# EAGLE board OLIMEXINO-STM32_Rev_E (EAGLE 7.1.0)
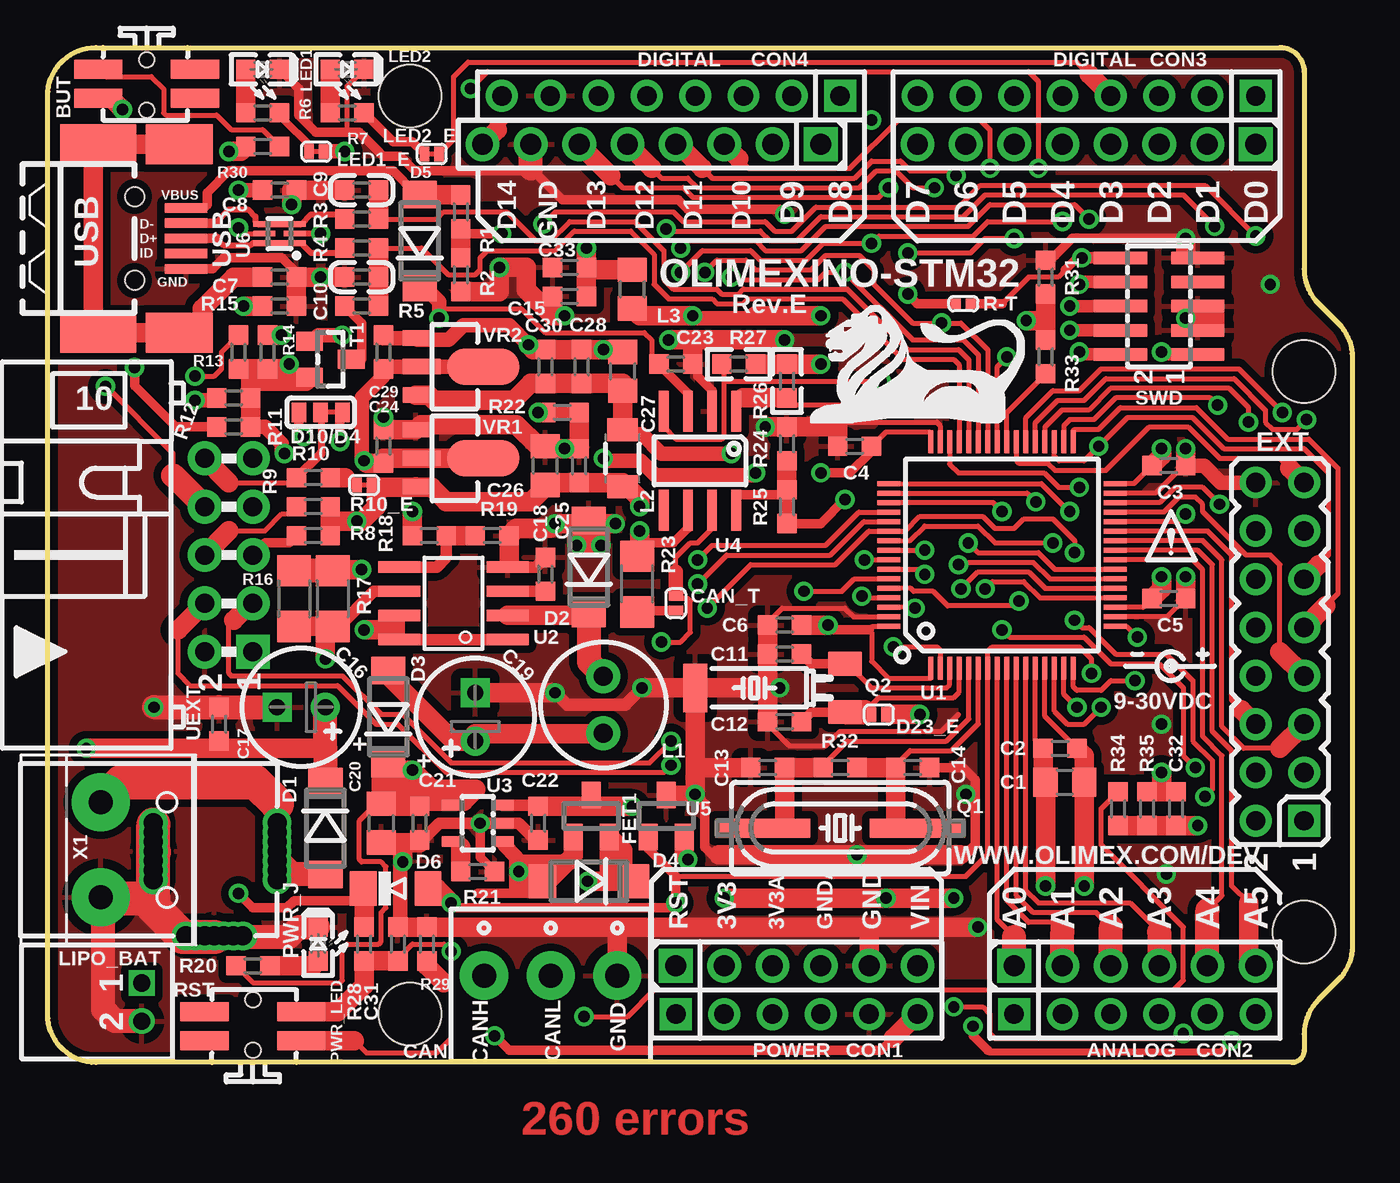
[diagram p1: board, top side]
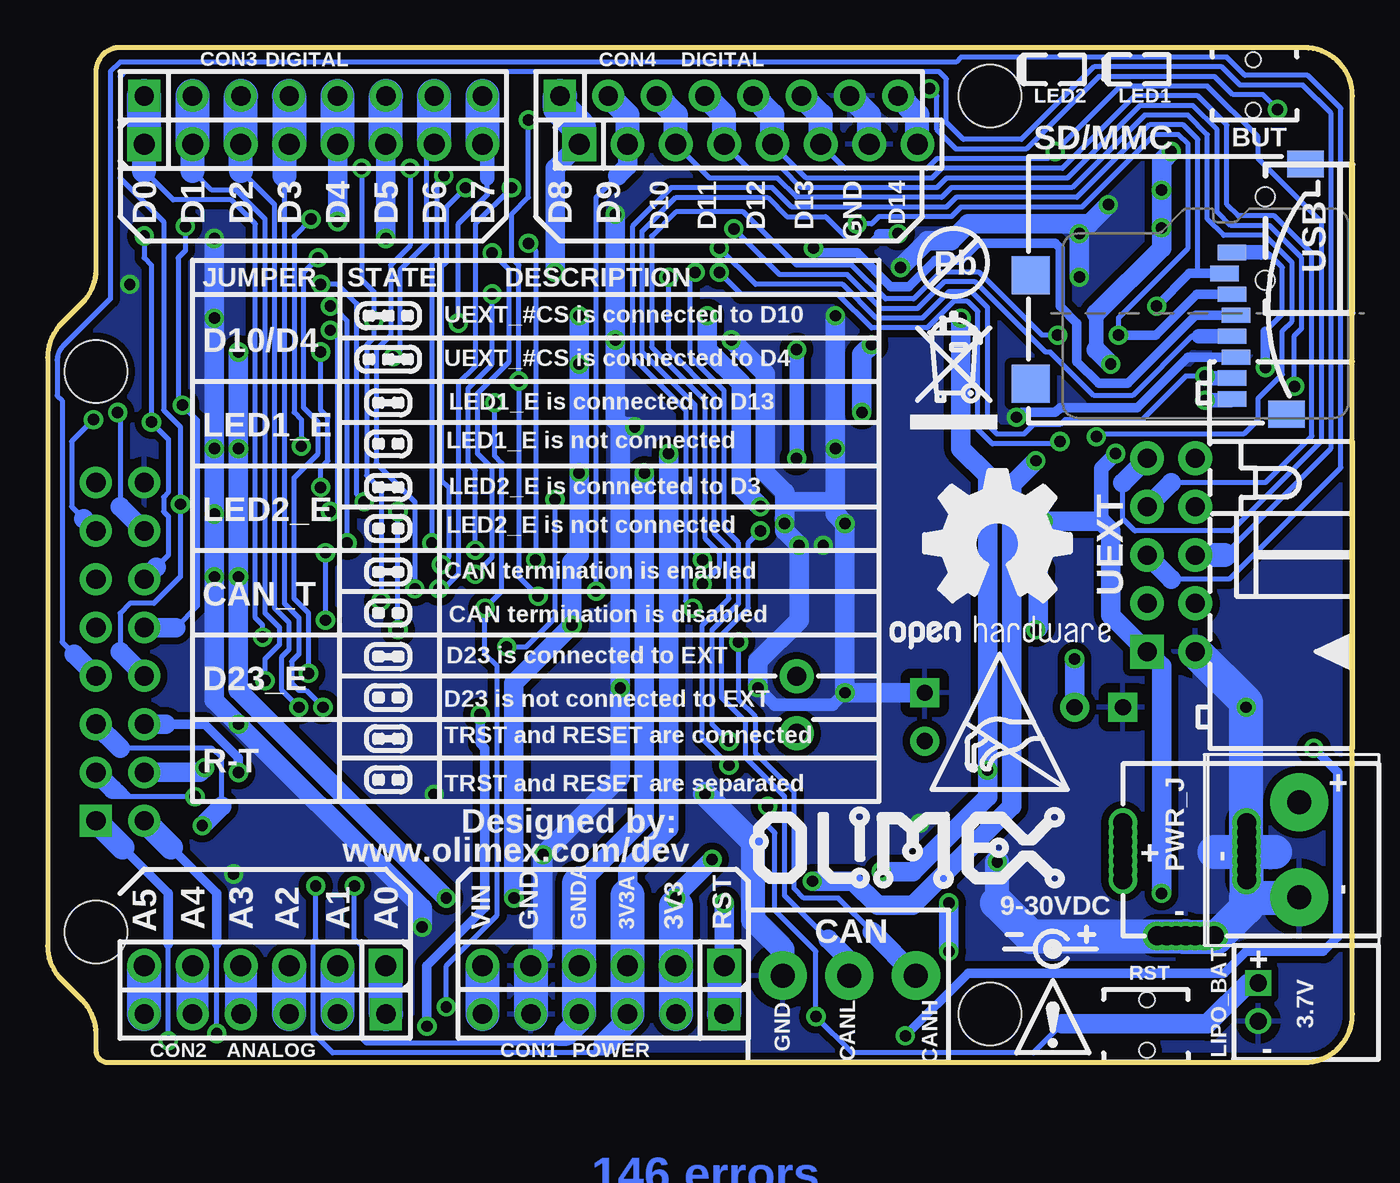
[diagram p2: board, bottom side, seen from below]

Size 68.58 x 53.34 mm. Coordinates in mm from the lower left corner, seen from the top.
Copper layers (1+16): Top 0.035mm / dielectric 1.5mm / Bottom 0.035mm
Design rules "default": minimum track width 10mil, minimum drill 0.6mm, track to track 9.5mil, track to pad 9.5mil, pad to pad 9.5mil, via to via 9.5mil, smd to smd 1mil, copper to edge 10mil, drill to drill 8mil, minimum pad ring 8mil, minimum via ring 8mil, stop-mask expansion 4mil, vias tented up to drill 25mil, thermal gap 20mil
Net classes: 0 default: width 0.241 mm, drill 0.584 mm, clearance 0.241 mm; 1 pwr: width 0.25 mm

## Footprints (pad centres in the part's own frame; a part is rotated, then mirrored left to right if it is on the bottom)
SW_TAKT3X4 = smd 2.54 x 1.016: 1_1 -2.54,0.762; 1_2 2.54,0.762; 2_1 -2.54,-0.762; 2_2 2.54,-0.762 | hole 0.8: 0,-1.397; 0,1.27
C0805_5MIL_DWS = smd 1.27 x 1.524: 1 -1.016,0; 2 1.016,0
C0603_DWS = smd 1.016 x 1.016: 1 -0.889,0; 2 0.889,0
C0603_DWS_NA = smd 1.016 x 1.016: 1 -0.889,0; 2 0.889,0
E2,5-6,3 = drill 0.864 pad 1.524: + -1.27,0 | drill 0.864 pad 1.524 square: - 1.27,0
CON3/3.5MM = drill 1.27 pad 2.54: 1 -1.75,-0.5; 2 1.75,-0.5; 3 5.25,-0.5
SJ_1_SMALLER = smd 0.508 x 0.762: 1 -0.381,0; 2 0.381,0
PN1X6 = drill 1.1 pad 1.778 square: 1 -6.35,0 | drill 1.1 pad 1.778: 2 -3.81,0; 3 -1.27,0; 4 1.27,0; 5 3.81,0; 6 6.35,0
PN1X8 = drill 1.1 pad 1.778 square: 1 -8.89,0 | drill 1.1 pad 1.778: 2 -6.35,0; 3 -3.81,0; 4 -1.27,0; 5 1.27,0; 6 3.81,0; 7 6.35,0; 8 8.89,0
MLL-41 = smd 1.45 x 1.8: A 2.445,0; K -2.445,0
MINI-MELF = smd 1.4 x 1.8: A 1.7,0; C -1.7,0
SJ_2_SMALL = smd 0.762 x 1.016: 1 -1.143,0; 2 0,0; 3 1.143,0
HN2X8-MALE = drill 1.016 pad 1.676 square: 1 -8.89,-1.27 | drill 1.016 pad 1.676: 2 -8.89,1.27; 3 -6.35,-1.27; 4 -6.35,1.27; 5 -3.81,-1.27; 6 -3.81,1.27; 7 -1.27,-1.27; 8 -1.27,1.27; 9 1.27,-1.27; 10 1.27,1.27; 11 3.81,-1.27; 12 3.81,1.27; 13 6.35,-1.27; 14 6.35,1.27; 15 8.89,-1.27; 16 8.89,1.27
SOT23 = smd 1 x 1.4: 1 -0.95,-1.1; 2 0.95,-1.1; 3 0,1.1
SW68 = drill 1 pad 1.778: 1 -1.5,0; 2 1.5,0
L3216C = smd 1.2 x 1.6: 1 -1.5,0; 2 1.5,0
L0805_5MIL_DWS = smd 1.27 x 1.524: 1 -1.016,0; 2 1.016,0
LED-0603 = smd 1.016 x 1.016: A 0.889,0; C -0.889,0
SJ_1_SMALLER_CLOSE = smd 0.508 x 0.762: 1 -0.381,0; 2 0.381,0
DW02R = drill 0.9 square: 1 -1,0 | drill 0.9: 2 1,0
STM32-MAPLE_PATFORM = drill 1.016 pad 1.676: 3V3 35.56,2.54; 3V3A 38.1,2.54; A1 53.34,2.54; A2 55.88,2.54; A3 58.42,2.54; A4 60.96,2.54; A5 63.5,2.54; D1 60.96,50.8; D2 58.42,50.8; D3 55.88,50.8; D4 53.34,50.8; D5 50.8,50.8; D6 48.26,50.8; D7 45.72,50.8; D9 39.116,50.8; D10 36.576,50.8; D11 34.036,50.8; D12 31.496,50.8; D13 28.956,50.8; D14 23.876,50.8; GND 43.18,2.54; GND@1 26.416,50.8; GNDA 40.64,2.54; VIN 45.72,2.54 | drill 1.016 pad 1.676 square: A0 50.8,2.54; D0 63.5,50.8; D8 41.656,50.8; RST 33.02,2.54 | hole 3.3: 66.04,36.322; 66.04,6.858; 19.05,50.8; 19.05,2.54
PWR_JACK_UNI_MILLING = drill 1: + 0,4.75; +1 0,5.25; +2 0,5.75; +3 0,6.25; +4 0,4.25; +5 0,3.75; +6 0,3.25; - -6.5,4.75; -1 -6.5,5.25; -2 -6.5,5.75; -3 -6.5,4.25; -4 -6.5,3.75; -5 -6.5,6.25; -6 -6.5,3.25; -- -3.3,0.3; --1 -3.8,0.3; --2 -4.3,0.3; --3 -4.8,0.3; --4 -2.8,0.3; --5 -2.3,0.3; --6 -1.8,0.3
HC49/SMD2_THIN = smd 5 x 1: 1 -4.064,0; 2 4.064,0
TC26H_3_REPAIR_SMD = smd 1.27 x 1.778: 1 -1.27,0; 2 1.27,0 | smd 2.54 x 1.27: GND 0,7.874
R0603_5MIL_DWS = smd 1.016 x 1.016: 1 -0.889,0; 2 0.889,0
R1206_5MIL_WS = smd 1.651 x 1.778: 1 -1.46,0; 2 1.46,0
0603_0R = smd 1.016 x 1.016: 1 -0.889,0; 2 0.889,0
R0603_5MIL_DWS_NA = smd 1.016 x 1.016: 1 -0.889,0; 2 0.889,0
SJ_1_THE_SMALLEST = smd 0.508 x 0.508: 1 -0.381,0; 2 0.381,0
TFR-MEM-CON = smd 0.8 x 1.5: 1 -3.2,10.7; 2 -2.1,10.3; 3 -1,10.7; 4 0.1,10.9; 5 1.2,10.7; 6 2.3,10.9; 7 3.4,10.7; 8 4.5,10.7 | smd 2 x 2: 9 3.7,0.1; 10 -2,0.1 | smd 1.4 x 1.9: 11 5.3,13.55; 12 -7.85,14.55
ML10_50MILS_M = smd 0.66 x 2.794: 1 -2.54,-2.032; 2 -2.54,2.032; 3 -1.27,-2.032; 4 -1.27,2.032; 5 0,-2.032; 6 0,2.032; 7 1.27,-2.032; 8 1.27,2.032; 9 2.54,-2.032; 10 2.54,2.032
SOT-23 = smd 1 x 1.4: 1 -0.95,-1.1; 2 0.95,-1.1; 3 0,1.1
LPTQFP64 = smd 1.2 x 0.254: 1 -5.95,3.75; 2 -5.95,3.25; 3 -5.95,2.75; 4 -5.95,2.25; 5 -5.95,1.75; 6 -5.95,1.25; 7 -5.95,0.75; 8 -5.95,0.25; 9 -5.95,-0.25; 10 -5.95,-0.75; 11 -5.95,-1.25; 12 -5.95,-1.75; 13 -5.95,-2.25; 14 -5.95,-2.75; 15 -5.95,-3.25; 16 -5.95,-3.75; 33 5.95,-3.75; 34 5.95,-3.25; 35 5.95,-2.75; 36 5.95,-2.25; 37 5.95,-1.75; 38 5.95,-1.25; 39 5.95,-0.75; 40 5.95,-0.25; 41 5.95,0.25; 42 5.95,0.75; 43 5.95,1.25; 44 5.95,1.75; 45 5.95,2.25; 46 5.95,2.75; 47 5.95,3.25; 48 5.95,3.75 | smd 0.254 x 1.2: 17 -3.75,-5.95; 18 -3.25,-5.95; 19 -2.75,-5.95; 20 -2.25,-5.95; 21 -1.75,-5.95; 22 -1.25,-5.95; 23 -0.75,-5.95; 24 -0.25,-5.95; 25 0.25,-5.95; 26 0.75,-5.95; 27 1.25,-5.95; 28 1.75,-5.95; 29 2.25,-5.95; 30 2.75,-5.95; 31 3.25,-5.95; 32 3.75,-5.95; 49 3.75,5.95; 50 3.25,5.95; 51 2.75,5.95; 52 2.25,5.95; 53 1.75,5.95; 54 1.25,5.95; 55 0.75,5.95; 56 0.25,5.95; 57 -0.25,5.95; 58 -0.75,5.95; 59 -1.25,5.95; 60 -1.75,5.95; 61 -2.25,5.95; 62 -2.75,5.95; 63 -3.25,5.95; 64 -3.75,5.95
SO-8 = smd 0.6 x 2.2: 1 -1.905,-2.854; 2 -0.635,-2.854; 3 0.635,-2.854; 4 1.905,-2.854; 5 1.905,2.854; 6 0.635,2.854; 7 -0.635,2.854; 8 -1.905,2.854
SOT-23-5 = smd 0.55 x 1.2: 1 -0.95,-1.3; 2 0,-1.3; 3 0.95,-1.3; 4 0.95,1.3; 5 -0.95,1.3
SO-08_THIN = smd 0.508 x 2.159: 1 -1.905,-2.603; 2 -0.635,-2.603; 3 0.635,-2.603; 4 1.905,-2.603; 5 1.905,2.603; 6 0.635,2.603; 7 -0.635,2.603; 8 -1.905,2.603
USBLC6-2P6 = smd 0.3 x 1.46: 1 -0.5,-0.65; 3 0.5,-0.65; 4 0.5,0.65; 6 -0.5,0.65 | smd 0.3 x 1.16: 2 0,-0.8; 5 0,0.8
BH10R = drill 1 pad 1.778 square: 1 -5.08,-1.27 | drill 1 pad 1.778: 2 -5.08,1.27; 3 -2.54,-1.27; 4 -2.54,1.27; 5 0,-1.27; 6 0,1.27; 7 2.54,-1.27; 8 2.54,1.27; 9 5.08,-1.27; 10 5.08,1.27
USB_MINI_9PIN = smd 2.25 x 0.5: D+ 2.706,0; D- 2.706,0.8; GND 2.706,-1.6; ID 2.706,-0.8; VBUS 2.706,1.6 | smd 4 x 2.1: GND1 -1.9,4.95; GND3 -1.9,-4.95 | smd 3.5 x 2.1: GND2 2.35,4.95; GND4 2.35,-4.95 | hole 1: 0,2.2; 0,-2.2
SOT89_REP_THERMALOFF = smd 0.8 x 1.4: 1 -1.499,-1.981; 3 1.499,-1.981 | smd 0.8 x 2: 2 0,-1.681 | smd 1.93 x 3.81: P$2 0,1.57
W237-102 = drill 1.27 pad 3.048: 1 -2.5,-1.27; 2 2.5,-1.27

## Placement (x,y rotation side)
BUT  SW-SIDE_WTCM-TR(3X4)  [SW_TAKT3X4]  5.21,51.44 0 top
C1  10uF/6.3V  [C0805_5MIL_DWS]  53.47,14.73 0 top
C2  100nF  [C0603_DWS]  53.21,16.51 0 top
C3  100nF  [C0603_DWS]  58.93,31.37 180 top
C4  100nF  [C0603_DWS]  42.42,32.38 0 top
C5  100nF  [C0603_DWS]  58.93,24.38 180 top
C6  4.7uF/6.3V  [C0603_DWS]  38.73,22.99 0 top
C7  10nF  [C0603_DWS]  12.19,41.27 0 top
C8  100nF  [C0603_DWS]  12.19,45.85 180 top
C9  NA(47pF)  [C0603_DWS_NA]  16.51,45.85 180 top
C10  NA(47pF)  [C0603_DWS_NA]  16.51,41.27 180 top
C11  10pF  [C0603_DWS]  38.73,21.46 180 top
C12  10pF  [C0603_DWS]  38.73,17.91 180 top
C13  27pF  [C0603_DWS]  37.85,15.49 180 top
C14  27pF  [C0603_DWS]  45.47,15.49 0 top
C15  22uF/6.3V  [C0603_DWS]  27.43,40.26 180 top
C16  CE 100uF/35V/6.3x11mm/RM2.5  [E2,5-6,3]  13.34,18.67 180 top
C17  100nF  [C0603_DWS]  9.02,17.78 90 top
C18  820pF  [C0603_DWS]  26.16,25.65 90 top
C19  CE 470uF/10V/6.3x11mm/RM2.5  [E2,5-6,3]  22.48,18.16 90 top
C20  10uF/6.3V  [C0805_5MIL_DWS]  17.53,12.57 270 top
C21  2.2uF  [C0603_DWS]  19.56,12.57 270 top
C22  2.2uF  [C0603_DWS]  25.78,12.57 270 top
C23  100nF  [C0603_DWS]  33.02,36.7 0 top
C24  2.2uF  [C0603_DWS]  17.65,32.38 90 top
C25  100nF  [C0603_DWS]  27.94,31.37 90 top
C26  10uF/6.3V  [C0805_5MIL_DWS]  26.16,31.37 90 top
C27  10uF/6.3V  [C0805_5MIL_DWS]  30.23,36.32 90 top
C28  10nF  [C0603_DWS]  28.07,36.58 90 top
C29  2.2uF  [C0603_DWS]  17.65,37.34 90 top
C30  2.2uF  [C0603_DWS]  26.16,36.58 90 top
C31  100nF  [C0603_DWS]  18.41,6.22 90 top
C32  10nF  [C0603_DWS]  59.31,13.34 270 top
C33  22uF/6.3V  [C0603_DWS]  27.43,41.78 180 top
CAN  TB3-3.5MM  [CON3/3.5MM]  28.19,4.06 180 top
CAN_T  Open  [SJ_1_SMALLER]  33.02,24.13 90 top
CON1  NA  [PN1X6]  39.37,5.08 0 top
CON2  NA  [PN1X6]  57.15,5.08 0 top
CON3  NA  [PN1X8]  54.61,48.26 180 top
CON4  NA  [PN1X8]  31.75,48.26 180 top
D1  1N5819S/SS14  [MLL-41]  14.61,12.32 270 top
D2  1N5819S/SS14  [MLL-41]  28.45,26.04 90 top
D3  1N5819S/SS14  [MLL-41]  17.91,18.16 90 top
D4  1N5819S/SS14  [MLL-41]  28.45,9.53 180 top
D5  1N5819S/SS14  [MLL-41]  19.56,43.18 90 top
D6  1N4148/mini-melf  [MINI-MELF]  18.29,9.14 0 top
D10/D4  D10:Open/D4:Close  [SJ_2_SMALL]  14.35,34.16 180 top
D23_E  Open  [SJ_1_SMALLER]  43.69,18.29 0 top
EXT  PN2x8  [HN2X8-MALE]  64.77,21.59 90 top
FET1  IRLML6402  [SOT23]  28.57,12.95 0 top
L1  CL10uH SW68  [SW68]  29.21,18.8 270 top
L2  NA  [L3216C]  30.23,31.75 90 top
L3  CL470nH/0805/1.76R/250mA  [L0805_5MIL_DWS]  30.73,40.64 90 top
LED1  GREEN(0603)  [LED-0603]  11.3,52.2 180 top
LED1_E  Close  [SJ_1_SMALLER_CLOSE]  14.12,47.88 0 top
LED2  YELLOW(0603)  [LED-0603]  15.75,52.2 180 top
LED2_E  Close  [SJ_1_SMALLER_CLOSE]  20.19,47.75 0 top
LIPO_BAT  DW02R  [DW02R]  4.95,3.17 270 top
PLATFORM1  STM32-MAPLE_PLATFORM  [STM32-MAPLE_PATFORM]  0,0 0 top
PWR_J  YDJ-1136  [PWR_JACK_UNI_MILLING]  12.06,6.35 0 top
PWR_LED  RED(0603)  [LED-0603]  14.22,6.22 270 top
Q1  Q8.000MHz/20pF/HC-49SM(SMD)  [HC49/SMD2_THIN]  41.66,12.32 180 top
Q2  32768Hz/6pF  [TC26H_3_REPAIR_SMD]  41.91,19.68 90 top
R1  15k  [R0603_5MIL_DWS]  21.72,44.7 270 top
R2  22k  [R0603_5MIL_DWS]  21.72,41.4 270 top
R3  22R  [R0603_5MIL_DWS]  16.51,44.32 180 top
R4  22R  [R0603_5MIL_DWS]  16.51,42.8 180 top
R5  1.5k  [R0603_5MIL_DWS]  16.51,39.75 180 top
R6  2k  [R0603_5MIL_DWS]  11.3,49.91 0 top
R7  2k  [R0603_5MIL_DWS]  15.75,49.91 0 top
R8  4.7k  [R0603_5MIL_DWS]  13.97,27.69 0 top
R9  4.7k  [R0603_5MIL_DWS]  13.97,29.21 0 top
R10  10k  [R0603_5MIL_DWS]  13.97,30.73 0 top
R10_E  Close  [SJ_1_SMALLER_CLOSE]  16.64,30.35 0 top
R11  100k  [R0603_5MIL_DWS]  9.78,33.4 180 top
R12  100k  [R0603_5MIL_DWS]  9.78,34.92 180 top
R13  100k  [R0603_5MIL_DWS]  10.03,37.34 90 top
R14  10k  [R0603_5MIL_DWS]  11.56,37.34 90 top
R15  1M  [R0603_5MIL_DWS]  12.19,39.75 180 top
R16  0.47R  [R1206_5MIL_WS]  12.95,24.38 90 top
R17  0.47R  [R1206_5MIL_WS]  14.99,24.38 90 top
R18  3.01k/1%  [R0603_5MIL_DWS]  20.07,27.69 0 top
R19  1k/1%  [R0603_5MIL_DWS]  23.37,27.69 0 top
R20  2k  [R0603_5MIL_DWS]  10.79,5.08 0 top
R21  15k  [R0603_5MIL_DWS]  22.61,10.03 180 top
R22  0R(boad mounted)  [0603_0R]  27.05,34.16 180 top
R23  120R  [R1206_5MIL_WS]  30.99,25.15 270 top
R24  10k  [R0603_5MIL_DWS]  38.86,32.51 270 top
R25  0R(boad mounted)  [0603_0R]  38.86,29.21 90 top
R26  NA(4.7k)  [R0603_5MIL_DWS_NA]  38.86,35.81 270 top
R27  NA(4.7k)  [R0603_5MIL_DWS_NA]  36.32,36.7 180 top
R28  10k  [R0603_5MIL_DWS]  16.64,6.22 270 top
R29  330R  [R0603_5MIL_DWS]  19.94,6.22 270 top
R30  1k  [R0603_5MIL_DWS]  11.3,48.13 0 top
R31  10k  [R0603_5MIL_DWS]  52.45,41.27 90 top
R32  1M  [R0603_5MIL_DWS]  41.66,15.49 180 top
R33  1k  [R0603_5MIL_DWS]  52.45,37.08 270 top
R34  3M  [R0603_5MIL_DWS]  56.26,13.34 90 top
R35  1M  [R0603_5MIL_DWS]  57.78,13.34 90 top
R-T  Open  [SJ_1_THE_SMALLEST]  48.13,39.88 0 top
RST  SW-SIDE_WTCM-TR(3X4)  [SW_TAKT3X4]  10.79,1.91 180 top
SD/MMC  MICRO  [TFR-MEM-CON]  17.02,39.37 270 bottom
SWD  GPH127SMT-02x05(PIN7-CUT)  [ML10_50MILS_M]  58.42,39.75 90 top
T1  DTA114YKA  [SOT-23]  14.86,36.96 270 top
U1  STM32F103RBT6(LQFP64)  [LPTQFP64]  50.16,26.67 90 top
U2  MC33063ADR(SO8)  [SO-8]  21.34,24.13 90 top
U3  MCP73812T-420I/OT  [SOT-23-5]  22.61,12.57 90 top
U4  MCP2551-I/SN  [SO-08_THIN]  34.29,31.62 180 top
U5  NA  [SOT23]  32.51,12.95 0 top
U6  NA  [USBLC6-2P6]  12.19,43.56 90 top
U$1  [LION_12X7MM]  45.34,35.18 0 top
U$5  [PB_SMALL]  20.95,42.04 0 bottom
U$6  [RECYCLE_BIN1/8]  23.24,33.27 0 bottom
U$7  [ESD_SYMBOL]  22.1,14.35 0 bottom
U$8  [ATTENTION_SMALL]  57.78,26.4 0 top
U$9  [OLIMEX1_V]  13.97,9.02 0 bottom
U$10  [ROHS]  not placed on the board
U$11  [LOGO-OPENHARDWARE_8X8]  18.67,27.18 0 bottom
U$12  [ATTENTION]  17.65,0.51 0 bottom
UEXT  BH10R  [BH10R]  9.53,26.67 90 top
USB  USB-MINI  [USB_MINI_9PIN]  4.57,43.31 0 top
VR1  MCP1700T-3302E/MB  [SOT89_REP_THERMALOFF]  21.34,31.75 270 top
VR2  MCP1700T-3302E/MB  [SOT89_REP_THERMALOFF]  21.34,36.58 270 top
X1  NA  [W237-102]  4.06,11.18 270 top

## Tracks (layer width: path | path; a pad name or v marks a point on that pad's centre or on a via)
+5V  (via drill 0.6)
  Top 0.254: R20.1 10.79,4.19 15.37,4.19 15.49,4.32 15.49,5.97 15.75,6.22 17.4,6.22 17.53,6.35 17.53,7.87 17.78,8.13 17.78,10.29 17.53,10.54 16.51,10.54 16.38,10.67 16.38,12.7 17.27,13.59 C20.1 | C23.1 31.75,37.08 31.75,37.97 31.37,38.35 26.16,38.35 24.89,39.62 20.57,39.62
  Top 0.508: U4.3 33.66,35.18 C23.1 | 22.61,8.89 24.86,8.89 24.86,9.14
  Top 0.559: U3.1 23.91,11.53 24,11.43
  Top 0.61: U3.4 19.56,13.52 C21.1
  Top 0.762: v24.77,10.03 24.64,10.03 24.64,10.54 | 24,11.43 24.64,10.79 24.64,10.54 | v20.57,39.12 20.57,39.62 20.57,39.97 19.81,40.73 D5.K | 24.64,10.54 27.3,10.54
  Top 1.016: v19.18,28.96 R18.1 | 17.91,15.37 D3.K 17.91,15.49 | 17.91,15.37 v19.18,15.37 20.32,14.22 | 17.53,13.72 C20.1 17.53,13.46 C21.1 19.56,13.72 17.53,13.72 | FET1.1 27.62,10.86 27.3,10.54 26.29,9.53 D4.A 26,10.03 v24.77,10.03 24.77,9.14 24.86,9.14 26,9.14 | 17.53,13.72 21.87,13.72 22.5,14.35 17.91,14.35 17.91,15.37 | 17.53,13.72 17.53,15.49 17.91,15.49 | 17.91,15.49 17.91,15.37
  Bottom 1.016: v24.77,10.03 23.11,10.03 19.18,13.97 v19.18,15.37 v19.18,28.96 19.18,30.86 20.57,32.26 v20.57,39.12
+5V_USB
  Top 0.508: USB.VBUS 8.2,44.91 8.38,45.09 8.38,45.72 9.53,46.86 18.16,46.86 19.3,45.72 19.56,45.72
  Top 0.762: 19.56,45.72 19.56,45.59
  Top 1.016: D5.A 19.56,45.59 R1.1
+24V  (via drill 0.6)
  Top 0.508: v23.5,1.4 24.26,0.64 43.81,0.64 44.45,1.27
  Top 0.61: U2.6 17.14,24.77 15.24,22.86 15.24,22.73
  Top 1.016: R17.1 14.99,22.73 | v14.61,21.21 14.61,22.73 15.24,22.73 15.24,22.67 R17.1 | R17.1 R16.1 | v2.03,16.51 9.02,16.51 | 9.02,16.51 14.61,16.51 | 44.45,1.27 PLATFORM1.VIN | 9.02,16.51 C17.1
  Top 1.27: D1.K 14.61,16.51 C16.+
  Bottom 0.508: v2.03,16.51 0.76,15.24 0.76,6.6 1.52,5.84 5.59,5.84 6.73,4.7 20.19,4.7 v23.5,1.4
  Bottom 1.016: C16.+ v14.61,21.21
  Bottom 1.778: PLATFORM1.VIN CON1.6
AGND  (via drill 0.6)
  Top 0.254: U1.12 51.91,16.92 C2.1
  Top 0.762: v37.21,30.99 37.21,30.86 31.93,30.86 31.17,31.62 29.21,31.62 v29.21,31.75 | C29.2 17.65,38.08 VR2.1 19.46,37.97 21.08,37.97 21.84,38.73 24.26,38.73 v25.27,37.72 | R22.2 28.07,34.16
  Top 1.016: C2.1 52.32,14.73 C1.1 v52.45,9.27 | C27.2 30.23,37.47 v29.21,37.47 C28.2 C30.2 25.53,37.47 v25.27,37.72 | v25.78,34.16 R22.2
  Bottom 0.254: 41.27,1.52 41.27,1.02 41.78,1.02 | 41.78,1.02 51.82,1.02 52.07,1.27 52.07,6.1 52.45,6.48 v52.45,9.27 | 41.78,1.02 41.78,1.52
  Bottom 0.762: v29.21,31.75 v29.21,37.47
  Bottom 1.016: 40.64,9.4 37.21,12.83 v37.21,30.99 | v25.27,37.72 25.78,37.21 v25.78,34.16
  Bottom 1.27: 41.27,1.52 40.64,2.16 PLATFORM1.GNDA
  Bottom 1.778: PLATFORM1.GNDA CON1.4 40.64,9.4
BOOT0  (via drill 0.6)
  Top 0.254: U1.60 45.37,24.92 45.52,24.77 46.54,24.77 47.3,24 50.8,24 v51.05,24.26 | v52.07,46.99 52.07,51.56 51.56,52.07 23.11,52.07 v22.23,51.18
  Top 1.016: 52.45,38.99 R33.1 | BUT.2_1 3.35,50.67 v3.94,50.09 | v51.44,38.99 52.45,38.99 | 52.45,38.99 R31.1
  Bottom 0.254: v51.05,24.26 51.05,30.1 51.82,30.86 51.82,37.72 51.44,38.1 v51.44,38.99 51.44,40.51 52.07,41.15 v52.07,46.99 | v3.94,50.09 4.71,50.86 6.29,50.86 7.24,51.82 13.34,51.82 17.14,48.01 20.83,48.01 21.84,49.02 21.84,50.8 v22.23,51.18
D0(RXD2)  (via drill 0.6)
  Top 0.254: U1.17 56.71,22.92 v57.28,22.35
  Bottom 0.254: v57.28,22.35 57.28,22.99 57.66,23.37 57.66,44.07 58.93,45.34 61.98,45.34 63.5,46.86
  Bottom 1.27: 63.5,46.86 CON3.1
  Bottom 1.778: CON3.1 PLATFORM1.D0
D1(TXD2)  (via drill 0.6)
  Top 0.254: U1.16 53.91,19.75 54.1,19.56 55.37,19.56 55.88,20.07 v57.15,20.07
  Bottom 0.254: v57.15,20.07 57.15,21.21 56.39,21.97 56.39,22.86 57.15,23.62 57.15,44.32 58.67,45.85 59.94,45.85 60.96,46.86
  Bottom 1.27: 60.96,46.86 CON3.2
  Bottom 1.778: CON3.2 PLATFORM1.D1
D2  (via drill 0.6)
  Top 0.254: U1.14 52.91,18.46 53.59,17.78 54.48,17.78 v55.37,18.67
  Bottom 0.254: v55.37,18.67 56.26,19.56 56.26,21.34 55.88,21.72 55.88,23.11 56.64,23.88 56.64,45.09 58.42,46.86
  Bottom 1.27: 58.42,46.86 CON3.3
  Bottom 1.778: CON3.3 PLATFORM1.D2
D3(LED2)  (via drill 0.6)
  Top 0.254: U1.15 53.41,19.36 v54.1,18.67 | LED2_E.2 21.34,48.51 21.34,51.82 22.1,52.58 54.1,52.58 54.74,51.94
  Top 1.016: 54.74,51.94 PLATFORM1.D3
  Bottom 0.254: v54.1,18.67 54.99,19.56 55.37,19.56 55.75,19.94 55.75,21.08 55.37,21.46 55.37,23.37 56.13,24.13 56.13,46.61
  Bottom 1.27: 56.13,46.61 56.13,48.01 CON3.4
  Bottom 1.778: PLATFORM1.D3 CON3.4
D4  (via drill 0.6)
  Top 0.254: v42.93,26.42 U1.57 | v53.34,44.2 49.4,44.2 48.64,43.43 43.69,43.43 v43.31,43.05 40.77,43.05 39.88,42.16 37.47,42.16 36.96,42.67 34.42,42.67 v33.27,41.53 | 15.37,34.16 14.35,34.16
  Top 0.508: v15.37,32.64 15.37,34.16 D10/D4.1
  Bottom 0.254: v42.93,26.42 42.93,42.67 v43.31,43.05 | v15.37,32.64 15.49,32.51 18.92,32.51 19.68,33.27 19.68,39.47 20.22,40.01 20.95,40.01 22.35,38.61 25.27,38.61 27.05,40.39 32.13,40.39 v33.27,41.53
  Bottom 1.016: v53.34,44.2 CON3.5
  Bottom 1.778: CON3.5 PLATFORM1.D4
D5  (via drill 0.6)
  Top 0.254: U1.58 45.84,25.92 v46.1,25.65 | v45.21,42.55 48.51,42.55 49.28,43.31 v50.8,43.31
  Bottom 0.254: v46.1,25.65 45.21,26.54 45.21,31.24 45.97,32 45.97,35.18 44.32,36.83 44.32,41.66 v45.21,42.55
  Bottom 1.016: v50.8,43.31 CON3.6
  Bottom 1.778: CON3.6 PLATFORM1.D5
D6  (via drill 0.6)
  Top 0.254: U1.41 49.91,36.57 v50.42,37.08
  Bottom 0.254: v50.42,37.08 50.04,37.47 50.04,41.66 48.64,43.05 48.64,47.88 CON3.7
  Bottom 1.778: CON3.7 PLATFORM1.D6
D7(TXD1)  (via drill 0.6)
  Top 0.254: U1.42 49.41,37.45 48.01,38.86 v46.99,38.86 45.47,38.86 43.43,40.89 43.43,41.66 42.67,42.42 40.89,42.42 40.13,41.66 37.21,41.66 36.7,42.16 35.18,42.16 v34.54,41.53 | v32.77,16.89 31.62,15.75 21.21,15.75 18.67,18.29 17.53,18.29 15.49,20.32 9.65,20.32 9.53,20.45 9.53,22.99 9.78,23.24
  Top 1.016: 9.78,23.24 10.67,24.13 UEXT.3
  Bottom 0.254: v46.99,38.86 46.99,44.07 45.47,45.59 45.47,46.48 | v34.54,41.53 34.8,41.27 34.8,37.08 33.02,35.31 33.02,28.07 32.26,27.3 32.26,24.13 33.66,22.73 33.66,17.78 v32.77,16.89
  Bottom 0.508: 45.47,48.01 CON3.8
  Bottom 0.762: 45.47,46.48 45.47,48.01
  Bottom 1.778: CON3.8 PLATFORM1.D7
D8(RXD1)  (via drill 0.6)
  Top 0.254: U1.43 48.91,37.19 48.13,37.97 45.47,37.97 v41.91,41.53 40.89,41.53 40.51,41.15 36.07,41.15 v35.94,41.27 | v32.77,15.62 32.38,15.24 20.95,15.24 18.41,17.78 17.27,17.78 15.24,19.81 7.49,19.81 6.86,20.45 6.86,22.73
  Top 1.016: 6.86,22.73 UEXT.4
  Bottom 0.254: v35.94,41.27 35.94,37.47 33.53,35.05 33.53,27.81 32.77,27.05 32.77,24.38 34.16,22.99 34.16,17.02 v32.77,15.62
  Bottom 1.016: v41.91,41.53 41.91,46.99 CON4.1
  Bottom 1.778: CON4.1 40.64,49.15 41.66,50.16 PLATFORM1.D8
D9  (via drill 0.6)
  Top 0.254: U1.59 42.4,25.42 41.74,24.77 v39.75,24.77
  Bottom 0.254: v39.75,24.77 39.75,45.47 38.61,46.61
  Bottom 1.016: 38.61,46.61 38.1,47.12 CON4.2
  Bottom 1.27: CON4.2 38.1,49.78 PLATFORM1.D9
D10(#SS1)  (via drill 0.6)
  Top 0.254: U1.20 52.16,24.42 51.31,25.27 49.66,25.27 v49.28,24.89 | v49.53,46.99 49.53,49.02 49.02,49.53 44.7,49.53 42.16,46.99 36.83,46.99 36.32,47.5
  Top 0.508: v13.46,32.89 13.21,33.15 D10/D4.3
  Top 1.016: CON4.3 36.32,47.5
  Bottom 0.254: v49.28,24.89 49.28,29.46 51.31,31.5 51.31,37.47 50.55,38.23 50.55,41.91 49.53,42.93 v49.53,46.99 | CON4.3 33.78,46.48 30.23,46.48 29.21,45.47 21.59,45.47 21.08,45.97 14.73,45.97 10.92,49.78 8.64,49.78 7.62,48.77 7.62,44.32 6.77,43.47 4.61,43.47 3.17,42.04 3.17,38.96 3.68,38.46 3.68,36.17 4.95,34.9 4.95,33.78 5.71,33.02 13.34,33.02 v13.46,32.89
  Bottom 1.27: CON4.3 35.56,49.78 PLATFORM1.D10
D11(MOSI1)  (via drill 0.6)
  Top 0.254: U1.23 52.95,25.92 52.07,26.8 48.9,26.8 v48.39,27.3 | v47.75,46.61 47.5,46.86 45.34,46.86 44.83,47.37 43.31,47.37 42.42,46.48 34.92,46.48 34.42,46.99 | v3.05,35.53 3.05,35.56 6.6,32 6.6,30.86
  Top 1.016: CON4.4 33.15,48.26 34.42,46.99
  Top 1.27: UEXT.8 6.6,30.86
  Bottom 0.254: v48.39,27.3 48.39,42.04 48.13,42.29 48.13,46.23 v47.75,46.61 | CON4.4 31.75,46.99 29.97,46.99 28.96,45.97 21.84,45.97 21.34,46.48 14.99,46.48 11.18,50.29 8.38,50.29 7.11,49.02 7.11,44.7 6.39,43.98 4.36,43.98 2.67,42.29 2.67,38.58 3.05,38.2 v3.05,35.53
  Bottom 1.27: CON4.4 33.02,49.78 PLATFORM1.D11
D12(MISO1)  (via drill 0.6)
  Top 0.254: U1.22 52.69,25.42 51.82,26.29 48.01,26.29 v47.88,26.16 | v46.61,45.97 45.47,45.97 44.58,46.86 43.56,46.86 42.67,45.97 34.16,45.97 33.66,46.48 32.26,46.48 31.75,46.99
  Top 1.016: CON4.5 31.75,46.99
  Bottom 0.254: v47.88,26.16 47.5,26.54 47.5,30.23 47.88,30.61 47.88,41.78 47.62,42.04 47.62,44.96 v46.61,45.97 | CON4.5 28.7,46.48 22.1,46.48 21.59,46.99 15.24,46.99 11.43,50.8 8.13,50.8 6.6,49.28 6.6,45.09 6.01,44.49 4.1,44.49 2.13,42.52 2.13,32.92 4.57,30.48 9.53,30.48
  Bottom 1.016: 9.53,30.48 UEXT.7
  Bottom 1.27: CON4.5 30.48,49.78 PLATFORM1.D12
D13(SCK1/LED1)  (via drill 0.6)
  Top 0.254: U1.21 52.42,24.92 51.56,25.78 48.9,25.78 v48.01,24.89 | v44.2,45.97 43.69,45.47 33.91,45.47 33.4,45.97 30.23,45.97 29.59,46.61
  Top 0.508: 14.73,47.88 LED1_E.2
  Top 0.762: v15.62,47.88 14.73,47.88
  Top 1.016: CON4.6 29.59,46.61
  Bottom 0.254: v48.01,24.89 47.75,24.89 46.99,25.65 46.99,35.69 46.1,36.58 46.1,44.07 v44.2,45.97 | CON4.6 26.67,46.99 22.35,46.99 21.84,47.5 16,47.5 v15.62,47.88 12.19,51.31 7.62,51.31 4.95,48.64 4.95,47.5 1.63,44.17 1.63,32.66 6.35,27.94 11.43,27.94 12.06,28.57 12.06,30.48
  Bottom 1.016: 12.06,30.48 UEXT.9
  Bottom 1.27: CON4.6 27.94,49.78 PLATFORM1.D13
D14(CANRX)  (via drill 0.6)
  Top 0.254: v42.8,24.51 42.89,24.42 U1.61 | 35.56,35.81 v43.81,35.81 | U4.4 32.38,33.4 33.02,32.77 35.43,32.77 35.56,32.89 35.56,35.81 | R27.2 35.56,36.58 35.56,35.81 | 23.62,49.02 24.13,49.53 v43.31,49.53
  Top 1.016: 23.62,49.02 CON4.8
  Bottom 0.254: v42.8,24.51 43.81,25.53 v43.81,35.81 43.81,41.91 44.2,42.29 44.2,44.58 43.31,45.47 v43.31,49.53
  Bottom 1.27: CON4.8 22.86,49.78 PLATFORM1.D14
D15(A0)
  Top 0.254: U1.8 49.91,7.49 50.8,6.6
  Top 1.27: CON2.1 50.8,6.6
  Bottom 1.778: PLATFORM1.A0 CON2.1
D16(A1)
  Top 0.254: U1.9 50.41,8.51 50.8,8.13 51.56,7.37 52.83,7.37 | 53.34,6.86 53.34,7.37 52.83,7.37 | 52.83,7.37 52.83,6.86
  Top 1.27: CON2.2 53.34,6.86
  Bottom 1.778: PLATFORM1.A1 CON2.2
D17(A2)
  Top 0.254: U1.10 50.91,8.78 51.82,7.87 55.12,7.87 55.88,7.11
  Top 1.27: CON2.3 55.88,7.11
  Bottom 1.778: PLATFORM1.A2 CON2.3
D18(A3)
  Top 0.254: U1.11 51.41,9.04 52.07,8.38 56.9,8.38 58.42,6.86
  Top 1.27: 58.42,6.86 CON2.4
  Bottom 1.676: CON2.4 PLATFORM1.A3
D19(A4)
  Top 0.254: U1.24 60.19,26.42 60.71,25.91 60.71,17.14 61.72,16.13 61.72,8.76 60.96,8
  Top 1.27: CON2.5 60.96,8
  Bottom 1.676: PLATFORM1.A4 CON2.5
D20(A5)
  Top 0.254: U1.25 60.46,26.92 61.21,26.16 61.21,17.4 62.23,16.38 62.23,9.27 63.12,8.38
  Top 1.016: CON2.6 63.12,5.46 63.12,8.38
  Bottom 1.778: PLATFORM1.A5 CON2.6
D21(CAN_CTRL)  (via drill 0.6)
  Top 0.254: U1.2 46.91,21.66 46.74,21.84 v44.45,21.84
  Top 0.508: v41.91,29.59 40.64,28.32 R25.1
  Bottom 0.254: v44.45,21.84 43.43,21.84 41.91,23.37 v41.91,29.59
D22
  Top 0.254: U1.3 47.41,19.86 47.24,19.68 43.31,19.68 42.04,20.95 Q2.2
  Top 0.508: Q2.2 40.13,20.95 C11.1
D23
  Top 0.254: U1.4 47.91,19.47 47.62,19.18 43.69,19.18 43.31,18.8 43.31,18.41
  Top 0.508: 42.93,18.41 43.31,18.41 D23_E.1 | Q2.1 40.13,18.41 C12.1
  Top 1.27: Q2.1 42.93,18.41
D23_EXT  (via drill 0.6)
  Top 0.381: 49.4,0.64 49.47,0.57 61.66,0.57 v62.23,1.14
  Top 0.508: 44.32,18.29 D23_E.2 | 49.4,0.64 48.64,1.4 v48.64,1.91
  Top 1.016: v45.85,18.29 44.32,18.29
  Bottom 0.254: v62.23,1.14 62.23,6.22
  Bottom 0.508: v48.64,1.91 48.64,5.08 45.59,8.13 45.59,16.51 45.85,16.76 v45.85,18.29 | 62.23,6.22 62.23,8.89 64.64,11.3
  Bottom 1.27: 64.64,11.3 EXT.1
D24(CANTX)  (via drill 0.6)
  Top 0.254: U1.62 45.55,23.92 v45.59,23.88 | v47.62,2.92 49.15,2.92 49.53,2.54 49.53,1.52 49.78,1.27 59.44,1.27 v59.69,1.52 | v45.09,34.67 44.58,34.16 43.31,34.16 42.93,34.54 39.24,34.54 R26.2 | U4.1 36.2,34.92 36.58,34.92
  Top 1.016: R26.2 36.58,34.92
  Bottom 0.254: v47.62,2.92 47.62,5.08 44.96,7.75 44.96,20.83 45.59,21.46 v45.59,23.88 44.7,24.77 44.7,31.5 45.09,31.88 v45.09,34.67 | v59.69,1.52 59.69,6.22
  Bottom 0.508: 59.69,6.22 59.69,8.89 62.1,11.3
  Bottom 1.27: 62.1,11.3 EXT.2
D25(MMC_CS)  (via drill 0.6)
  Top 0.254: v53.98,26.8 53.98,27.43 52.83,28.57 51.31,28.57 50.8,28.07 49.78,28.07 49.15,28.7 45.85,28.7 45.06,27.92 U1.54 43.16,27.92 41.4,26.16 36.96,26.16 v34.67,23.88 | v53.98,23.24 54.36,22.86 54.74,22.86 56.13,21.46 58.8,21.46 60.2,20.07 60.2,16.89 61.21,15.88 61.21,14.35 v60.83,13.97
  Top 1.016: v10.29,39.75 R15.2
  Bottom 0.254: v53.98,26.8 v53.98,23.24 | v60.83,13.97 64.24,13.97 | 64.24,13.97 64.39,13.97 | 64.39,13.97 65.15,13.97 65.15,14.35 | v34.67,23.88 35.05,24.26 35.05,34.29 37.85,37.08 37.85,43.94 35.81,45.97 30.48,45.97 29.46,44.96 21.34,44.96 20.83,45.47 14.48,45.47 10.67,49.28 8.89,49.28 8.13,48.51 8.13,41.47 | 64.39,13.97 64.77,14.35 | 64.24,13.97 64.75,14.48
  Bottom 0.508: SD/MMC.2 8.13,41.47 8.57,41.47 v10.29,39.75
  Bottom 1.016: 65.15,14.35 EXT.3
D26  (via drill 0.6)
  Top 0.254: U1.51 49.7,29.42 v50.16,28.96 | v50.16,22.73 50.55,22.35 54.48,22.35 55.88,20.95 58.42,20.95 59.69,19.68 59.69,16.13 v60.33,15.49
  Bottom 0.254: v50.16,22.73 v50.16,28.96
  Bottom 1.016: v60.33,15.49 60.58,15.24 EXT.4
D27  (via drill 0.6)
  Top 0.254: U1.26 60.72,27.42 61.72,26.42 61.72,17.65 62.87,16.51 64.77,16.51
  Top 1.016: EXT.5 64.77,16.51 | R34.1 R35.1 C32.2 v60.45,12.45
  Bottom 0.254: 59.44,13.46 59.44,16 59.94,16.51 64.77,16.51
  Bottom 1.016: v60.45,12.45 59.44,13.46 | 64.77,16.51 EXT.5
D28  (via drill 0.6)
  Top 0.254: U1.27 60.98,27.92 62.23,26.67 62.23,19.05 62.74,18.54
  Top 1.016: EXT.6 62.74,18.54 | R35.2 57.91,14.22 | 57.91,14.22 C32.1 | 57.91,14.22 58.55,14.22 v58.55,15.24
  Bottom 0.508: v58.55,15.24 58.55,16 60.33,17.78 62.36,17.78
  Bottom 1.016: 62.36,17.78 EXT.6
D29(SCL2)
  Top 0.254: U1.29 58.66,28.92 59.46,29.72 60.33,29.72 60.71,29.34 60.71,28.96 62.99,26.67 64.26,26.67 64.77,26.16 64.77,21.59
  Top 0.508: UEXT.5 11.43,27.3 12.7,27.3 R8.1
  Top 1.016: EXT.7 64.77,21.59
  Bottom 0.254: 67.18,21.46 67.82,22.1 67.82,34.8 68.07,35.05 68.07,36.92 arc45 67.77,37.64 65.28,40.13 65.28,52.07 64.77,52.58 20.83,52.58 20.57,52.83 6.6,52.83 5.65,51.88 2.35,51.88 0.61,50.14 0.61,31.27 6.48,25.4 9.53,25.4
  Bottom 1.016: 67.18,21.46 EXT.7 | 9.53,25.4 UEXT.5
D30(SDA2)  (via drill 0.6)
  Top 0.254: 9.53,27.94 11.43,27.94 12.32,28.83 12.7,28.83 R9.1 | U1.30 58.45,29.42 59.26,30.23 60.71,30.23 v61.59,29.34
  Top 1.016: UEXT.6 9.53,27.94
  Bottom 0.254: 64.77,21.59 64.77,23.62 64.26,24.13 62.99,24.13 61.59,25.53 v61.59,29.34 61.59,33.4 62.48,34.29 62.48,44.2 64.77,46.48 64.77,51.82 64.52,52.07 21.72,52.07 21.34,51.69 21.34,49.4 20.45,48.51 17.4,48.51 13.59,52.32 6.86,52.32 5.91,51.37 2.6,51.37 1.12,49.89 1.12,32.28 6.73,26.67
  Bottom 1.016: 64.77,21.59 EXT.8
  Bottom 1.27: 6.73,26.67 UEXT.6
D31(#SS2)
  Top 0.254: U1.33 53.91,33.21 53.98,33.27 55.24,33.27 56.39,34.42 60.38,34.42 62.03,32.77 66.29,32.77 67.82,31.24 67.82,24.64 67.18,24
  Top 1.016: 67.18,24 EXT.9
D32(SCK2)  (via drill 0.6)
  Top 0.254: U1.34 53.41,33.48 53.72,33.78 54.99,33.78 56.13,34.92 61.11,34.92 v61.49,34.54 | v61.34,43.94 59.69,45.59 49.28,45.59 48.13,44.45 40.64,44.45 39.37,43.18 37.97,43.18 37.47,43.69 32.64,43.69 v32.51,43.81
  Bottom 0.254: 61.85,22.86 60.71,24 60.71,33.76 v61.49,34.54 61.72,34.77 61.72,42.29 61.34,42.67 v61.34,43.94 | 8.08,38.18 8.43,38.18 11.56,35.05 13.59,35.05 15.88,37.34 16.13,37.34 19.81,41.02 21.46,41.02 22.86,39.62 24.77,39.62 26.54,41.4 30.1,41.4 v32.51,43.81
  Bottom 0.762: SD/MMC.5 8.08,38.18
  Bottom 1.016: 61.85,22.86 EXT.10
D33(MISO2)  (via drill 0.6)
  Top 0.254: U1.35 52.91,31.87 53.16,31.62 54.48,31.62 v55.24,32.38 56.77,33.91 60.17,33.91 61.82,32.26 66.04,32.26 67.31,30.99 67.31,26.67 66.8,26.16 | v54.74,44.32 53.98,45.09 49.53,45.09 48.39,43.94 40.89,43.94 39.62,42.67 37.72,42.67 37.21,43.18 33.66,43.18 v33.27,42.8 | R13.2 9.14,37.34 9.14,36.45 8.76,36.07 v7.75,36.07
  Top 1.016: 66.8,26.16 EXT.11
  Bottom 0.254: v55.24,32.38 55.24,33.78 55.63,34.16 55.63,43.43 v54.74,44.32 | v7.75,36.07 8.76,36.07 11.05,33.78 15.11,33.78 15.37,33.53 16.76,33.53 17.27,33.02 18.67,33.02 19.18,33.53 19.18,39.67 20.02,40.51 21.21,40.51 22.61,39.12 25.02,39.12 26.8,40.89 31.37,40.89 v33.27,42.8
  Bottom 0.508: 7.78,36.1 v7.75,36.07
  Bottom 0.762: SD/MMC.7 7.65,35.97 7.78,36.1
D34(MOSI2)  (via drill 0.6)
  Top 0.254: U1.36 52.41,33.39 53.31,34.29 54.71,34.29 55.85,35.43 62.1,35.43 63.12,34.42 v63.12,33.66 | v63.5,43.43 60.83,46.1 49.02,46.1 47.88,44.96 40.39,44.96 39.12,43.69 38.23,43.69 37.72,44.2 33.4,44.2 32.89,44.7 26.67,44.7 v26.04,44.07
  Top 1.016: v12.29,38.23 R14.2
  Bottom 0.254: 62.87,26.04 62.23,26.67 62.23,28.7 62.48,28.96 62.48,29.72 62.23,29.97 62.23,32.77 v63.12,33.66 63.12,41.91 63.5,42.29 v63.5,43.43 | v26.04,44.07 25.27,44.07 24.89,44.45 21.08,44.45 20.57,44.96 14.22,44.96 10.41,48.77 9.14,48.77 8.64,48.26 8.64,42.8 12.29,39.14 v12.29,38.23
  Bottom 0.508: SD/MMC.3 8.2,40.37 10.34,38.23 v12.29,38.23
  Bottom 1.016: 62.87,26.04 EXT.12
D35  (via drill 0.6)
  Top 0.254: U1.37 51.91,33.63 53.09,34.8 54.48,34.8 55.63,35.94 62.36,35.94 64.01,34.29 64.01,33.66 64.39,33.27 65.66,33.27 v66.17,33.78
  Bottom 0.254: v66.17,33.78 67.31,32.64 67.31,29.21 66.67,28.57
  Bottom 1.016: 66.67,28.57 EXT.13
D36  (via drill 0.6)
  Top 0.254: U1.38 51.41,33.89 52.83,35.31 54.23,35.31 55.37,36.45 62.61,36.45 v64.9,34.16
  Bottom 0.254: v64.9,34.16 64.77,34.04 64.77,29.21
  Bottom 1.016: 64.77,29.21 EXT.14
D37
  Top 0.254: U1.39 50.91,31.64 51.05,31.5 52.58,31.5 52.96,31.11 55.63,31.11 57.91,33.4 59.94,33.4 61.59,31.75 64.77,31.75 65.28,31.24
  Top 1.016: 65.28,31.24 EXT.15
D+
  Top 0.305: 8.89,43.31 9.25,42.95 10.68,42.95 10.79,43.06 U6.6 U6.1 13.33,43.06 13.84,42.55 15.62,42.55 R4.2
  Top 0.508: USB.D+ 8.89,43.31
D-
  Top 0.305: 8.8,44.11 9.53,44.83 10.54,44.83 10.92,44.45 10.92,44.2 11.06,44.06 U6.4 U6.3 13.33,44.06 13.84,44.58 15.62,44.58 R3.2
  Top 0.508: USB.D- 8.8,44.11
DISC  (via drill 0.6)
  Top 0.254: U1.53 42.9,28.42 41.15,26.67 35.69,26.67 v34.16,25.15 | T1.1 13.91,37.91
  Top 0.762: v15.49,38.23 14.23,38.23 13.91,37.91
  Bottom 0.254: v15.49,38.23 16.31,38.23 19.61,41.53 21.67,41.53 23.06,40.13 24.54,40.13 26.31,41.91 29.21,41.91 32,44.7 35.56,44.7 36.83,43.43 36.83,37.59 34.04,34.8 34.04,27.56 33.27,26.8 33.27,26.04 v34.16,25.15
GND  (via drill 0.6)
  Top 0.254: C12.2 37.85,17.78 38.99,16.64 40.89,16.64 41.66,17.4 46.99,17.4 47.88,18.29 | U1.63 42.37,23.42 41.91,23.88 38.61,23.88 37.85,23.11 C6.1 | U1.18 58.85,23.42 C5.1 | U1.31 58.24,29.92 59.31,30.99 59.44,30.99 C3.1 | U1.28 59.41,28.42 v59.82,28.83 | C4.1 41.53,33.66 46.74,33.66 46.91,33.48 U1.47 | LED2.C 15.75,51.31 15.75,48.9
  Top 0.305: v14.35,43.56 U6.2
  Top 0.508: R21.1 22.73,10.79 v22.73,12.57 | v34.04,14.1 34.54,13.59 34.54,11.3 34.92,10.92 35.28,10.92 | 47.95,10.92 48.26,10.92 48.77,11.43 48.77,14.86 48.13,15.49 C14.2 | 60.45,39.12 SWD.3 | 60.2,39.12 60.45,39.12 | 60.45,39.12 SWD.5 | U4.2 34.92,35.31 34.16,36.07 34.16,36.7 C23.2 | USB.GND 8.69,41.71 9.27,42.29 12.32,42.29 13.08,41.53 C7.2 | LED1.C 13.21,51.18 13.21,49.78 14.1,48.9 15.75,48.9 16.38,48.9 17.65,47.62 18.54,47.62 19.3,46.86 25.4,46.86 25.4,46.99 27.05,45.34 33.15,45.34 33.66,44.83 38.48,44.83 v38.73,44.58 | R31.2 52.7,42.42 52.96,42.42 53.85,43.31 v59.82,43.31 | C24.2 v17.65,33.91
  Top 0.61: 24.26,26.04 U2.4 | 24.26,26.04 25.65,26.04 C18.2 | C21.2 19.68,11.68 20.57,12.57 v22.73,12.57 U3.2 24.77,12.57 25.65,11.68 C22.2 | 24.26,26.42 24.26,26.04 | 59.82,42.55 59.82,42.29 SWD.9
  Top 0.66: v26.67,19.43 27.3,18.8 30.35,18.8 v31.24,19.68
  Top 0.762: 18.54,7.11 18.54,10.41 v18.67,10.54 | EXT.16 61.67,30.48 60.78,31.37 C3.1
  Top 1.016: C21.2 19.56,11.56 18.67,11.56 | C31.2 18.54,7.11 R29.1 29.94,7.11 | v18.67,10.54 18.67,11.56 | 18.67,11.56 C20.2 | 24.26,26.42 R19.2 24.64,28.07 26.42,28.07 v26.67,28.32 27.81,28.32 | v26.67,19.43 C19.- | 29.94,7.11 CAN.1 | C24.2 17.65,33.25 VR1.1 19.63,33.53 24.64,33.53 25.78,32.38 C26.2 26.16,32.26 v27.18,32.26 C25.2 R22.1 | 37.85,19.68 C12.2 | 37.85,19.68 C11.2 C6.1 | Q2.GND 37.85,19.68 | 34.04,15.49 C13.2 | 34.04,15.49 Q2.GND | U5.3 34.04,14.05 v34.04,14.1 34.04,15.49 | 47.95,10.92 v42.55,10.92 35.28,10.92 | 29.94,7.11 43.05,7.11 | 43.05,7.11 43.18,7.11 CON1.5 | v59.82,25.53 C5.1 | v59.82,32.26 C3.1 | v59.82,39.12 60.2,39.12 61.34,39.12 | 61.34,39.12 61.34,38.73 | 61.34,39.12 61.34,39.5 | v59.82,43.31 59.82,42.55 | Q2.GND v31.24,19.68 | 43.05,7.11 v48.9,7.11 | C10.2 v14.35,41.27 C7.2 R15.1 | 12.83,45.85 C8.1 | v12.83,45.09 12.83,45.85 | 12.83,45.85 C9.2 | v38.73,37.97 33.91,37.97 | 33.91,37.97 C23.2 | v37.72,33.4 R24.1 41.53,33.4 C4.1 | R2.2 23.75,40.51 v23.75,41.78 25.17,41.78 25.17,40.62 26.54,39.24 v27.18,39.24 | v38.48,19.68 37.85,19.68 | 33.91,37.97 v32.64,37.97 | 28.45,28.32 D2.A | 29.08,28.32 28.45,28.32 | 29.08,28.32 v29.84,28.32 | 27.81,28.32 28.45,28.32 | 27.81,28.32 v27.81,27.18 28.45,27.18 | 29.08,28.32 v29.08,27.18 28.45,27.18 | 28.45,27.18 28.45,28.32
  Top 1.27: 2.79,8.64 X1.2 2.92,8.68 2.92,2.79 3.54,2.17 LIPO_BAT.2 | PWR_LED.C 13.21,7.11 12.7,6.6 8.76,6.6 PWR_J.-- | v5.59,18.67 C17.2 C16.- | 25.4,46.99 CON4.7
  Top 1.778: 5.57,8.64 5.57,11.05 | 2.79,8.64 5.57,8.64 | 5.57,8.64 5.57,8.15 7.11,6.6 8.76,6.6 | 5.57,12.5 PWR_J.- 5.57,11.05 | 5.57,11.05 5.59,11.05
  Bottom 0.508: SD/MMC.6 8.65,37.07 11.3,34.42 15.37,34.42 15.62,34.16 17.4,34.16 v17.65,33.91
  Bottom 0.66: v26.67,19.43 27.3,18.8 30.35,18.8 v31.24,19.68
  Bottom 1.016: v59.82,43.31 v59.82,39.12 v59.82,32.26 v59.82,28.83 v59.82,25.53 59.82,19.05 48.9,8.13 v48.9,7.11 | CON1.5 42.55,5.71 v42.55,10.92 38.48,14.99 v38.48,19.68 38.48,33.4 v37.72,33.4 38.35,33.4 38.73,33.78 v38.73,37.97 v38.73,44.58 | 14.35,44.07 v14.35,43.56 v14.35,41.27 | 14.35,44.07 13.84,44.07 v12.83,45.09 | 27.18,29.46 27.18,28.83 v26.67,28.32 v26.67,19.43 C19.- | 27.18,29.46 v27.18,32.26 v27.18,39.24 | v23.75,41.78 22.35,43.18 21.08,43.18 20.19,44.07 14.35,44.07 | v32.64,37.97 30.86,36.2 30.86,30.99 29.84,29.97 29.84,29.46 | 29.84,29.46 v29.84,28.32 29.84,27.94 v29.08,27.18 29.08,23.24 31.24,21.08 v31.24,19.68 | 29.84,29.46 27.18,29.46
  Bottom 1.27: v5.59,18.67 5.59,18.92 | 5.59,11.3 5.57,11.3 | 18.67,8.38 v18.67,10.54 | CON4.7 25.4,49.78 PLATFORM1.GND@1 | CAN.1 29.94,5.94 31.5,7.49 31.5,11.56 v34.04,14.1
  Bottom 1.778: 5.59,18.92 UEXT.2 | 5.59,11.05 5.59,11.3 | 5.59,11.05 v5.59,18.67 | CON1.5 PLATFORM1.GND | 4.06,11.05 5.59,11.05 | 5.59,11.05 7.24,11.05 | 18.67,8.38 16.89,6.6 8.89,6.6 | PWR_J.-- 8.81,6.6 8.89,6.6 | 7.11,6.6 5.57,8.15 | 5.57,8.64 5.57,8.13 | 5.57,8.64 5.57,10.54 | 8.89,6.6 7.24,6.6 | 5.57,8.64 5.59,8.64 | 2.67,8.64 5.57,8.64
  other vias: 64.26,40.89 58.55,17.78 58.8,9.91 48.26,14.1
  pour Bottom (isolate 0.381, rank 2): -4.32,57.78 71.37,57.78 71.37,-6.48 -4.32,-6.48
  pour Top (isolate 0.406, rank 2): -3.43,57.15 70.87,57.15 70.87,-4.57 -3.43,-4.57
MCIDAT1  (via drill 0.6)
  Top 0.762: v7.75,34.8 8.76,34.8 R12.2
  Bottom 0.762: SD/MMC.8 6.39,34.8 v7.75,34.8
MCIDAT2  (via drill 0.6)
  Top 0.508: v4.57,36.52 4.57,35.56 6.73,33.4 R11.2
  Bottom 0.254: 4.22,42.32 3.68,41.78 3.68,39.32 4.57,38.43 | 4.22,42.32 4.57,42.67 4.83,42.67 4.83,42.57 | 4.22,42.32 4.8,42.32
  Bottom 0.508: v4.57,36.52 4.57,38.43
  Bottom 0.762: 4.83,42.57 SD/MMC.1
MMC_PWR  (via drill 0.6)
  Top 1.016: 28.32,41.66 C15.1 | v28.32,42.8 C33.1 28.32,41.66 | 28.32,41.66 L3.2
  Bottom 0.508: SD/MMC.4 8.23,39.27 11.81,35.69 13.34,35.69 14.48,36.83 14.48,38.86 15.37,39.75 15.37,42.8 15.62,43.05 19.68,43.05 20.57,42.16 21.92,42.16 23.32,40.77 24.26,40.77 26.04,42.55 28.07,42.55 v28.32,42.8
N$1
  Top 0.254: R23.2 30.99,23.75
  Top 0.508: 30.99,23.75 CAN_T.1
N$2
  Top 0.406: LED1_E.1 13.74,48.23 12.45,49.53 12.45,49.66 R6.2
N$3
  Top 0.508: R25.2 38.86,29.84 36.2,29.84 U4.8
  Top 1.016: R25.2 R24.2
N$4
  Top 0.508: R10_E.1 16.03,30.35 15.65,30.73
  Top 1.016: 15.65,30.73 R10.2
N$5
  Top 1.016: R7.1 LED2.A
N$6
  Top 0.508: LED2_E.1 19.18,48.39 18.16,48.39 R7.2
N$7
  Top 1.016: D3.A 17.91,20.32 21.34,16.89 C19.+ 22.48,17.27 29.19,17.27 L1.2
N$8
  Top 1.016: PWR_LED.A 13.97,5.08 R20.2
N$11
  Top 0.254: 16.13,1.14 16.76,0.51 20.45,0.51 21.21,1.27 21.21,4.19 20.83,4.19
  Top 1.016: RST.1_1 16.13,1.14 | 20.83,4.19 19.94,5.08 R29.2
N$12
  Top 0.254: BUT.1_1 3.05,51.82 5.46,51.82 6.1,51.18 6.1,49.91 6.22,49.78 8.89,49.78 9.65,49.02 11.3,49.02 R30.2
N$13
  Top 1.27: D1.A 14.61,9.91 12.83,9.91 12.06,10.67 12.06,11.05 PWR_J.+ 12.06,13.59
  Top 1.778: X1.1 3.85,14.73 10.92,14.73 12.06,13.59
N$22
  Top 0.559: U3.5 21.72,11.62 21.72,11.3
  Top 1.016: R21.2 21.72,11.3
N$23
  Top 1.016: R6.1 LED1.A
N$33
  Top 0.61: U2.3 C18.1
N$34  (via drill 0.6)
  Top 0.762: VR2.P$2 VR2.2 17.65,36.58 C29.1 17.65,36.07 16.51,34.92 16.51,31.75 v16.64,31.62
  Top 1.016: 30.23,9.53 D4.K | v28.38,9.53 29.52,9.53 | 29.52,9.53 FET1.2 30.23,11.15 30.23,9.53 | VR1.P$2 VR1.2 17.65,31.75 C24.1 16.76,31.5 v16.64,31.62 | 29.52,9.53 30.23,9.53 | 29.52,9.53 29.08,9.53
  Bottom 1.016: v28.38,9.53 26.22,9.53 24.95,8.26 23.11,8.26 17.91,13.46 17.91,30.35 v16.64,31.62
N$41
  Top 0.254: U1.5 48.41,18.06 47.24,16.89 42.04,16.89 40.77,15.62 R32.2
  Top 1.016: Q1.2 38.73,12.32 C13.1 R32.2
N$42
  Top 0.254: U1.6 48.91,17.8 47.5,16.38 45.34,16.38 44.58,15.62 C14.1
  Top 1.016: R32.1 C14.1 44.58,12.32 Q1.1
N$56
  Top 0.508: T1.3 16.51,36.96 16.51,38.86 R5.2
N$61
  Top 0.61: U2.5 20.45,26.04 20.95,26.54 R18.2
  Top 1.016: R18.2 R19.1
N$64  (via drill 0.6)
  Top 0.61: 18.48,22.73 U2.8 U2.1 | 18.1,22.73 18.48,22.73 | 18.48,22.73 U2.7
  Top 1.016: R17.2 14.99,25.91 v16.51,25.91 | v16.64,22.73 18.1,22.73
  Top 1.27: R17.2 R16.2
  Bottom 1.016: v16.64,22.73 16.51,22.86 v16.51,25.91
N$67
  Top 0.61: 28.45,23.5 D2.K
  Top 1.016: U2.2 28.45,23.5
  Top 1.27: 28.45,23.5 28.45,21.06 L1.1
N$76  (via drill 0.6)
  Top 0.254: R23.1 30.99,26.67 31.11,26.67
  Top 0.508: U4.6 33.66,28.07 32.89,27.3 31.11,27.3
  Top 1.016: v31.11,27.94 31.11,27.3 31.11,26.67
  Bottom 0.254: 27.56,6.48 29.84,8.76 29.84,13.97 31.88,16 31.88,17.91 33.15,19.18 33.15,22.48 31.75,23.88 31.75,27.3 v31.11,27.94
  Bottom 1.016: CAN.2 26.44,5.36 27.56,6.48
N$77  (via drill 0.6)
  Top 0.254: U4.7 34.92,28.07 34.16,27.3 33.78,27.3 33.02,26.54 33.02,25.78 | 33.02,24.64 33.15,24.64 33.4,24.38 33.66,24.38 33.78,24.26 33.78,22.61 33.27,22.1 v32.26,22.1
  Top 0.508: 33.02,24.64 CAN_T.2
  Top 0.762: 33.02,24.64 33.02,25.78
  Bottom 0.254: 25.24,6.86 27.02,8.64 28.83,8.64 29.34,9.14 29.34,14.22 31.37,16.26 31.37,18.16 32.26,19.05 v32.26,22.1
  Bottom 1.016: CAN.3 25.24,6.86
N$82
  Top 0.254: U1.40 50.41,34.16 R33.2
RESET  (via drill 0.6)
  Top 0.254: C31.1 18.41,5.46 19.18,6.22 20.83,6.22 v21.21,5.84 | 33.02,9.78 48.26,9.78 49.41,10.93 U1.7 49.41,21.6 49.66,21.84 54.23,21.84 54.86,21.21 v54.86,20.45 | v54.36,42.29 54.13,42.29 | 53.49,41.66 53.11,41.27 51.56,41.27 50.16,39.88
  Top 0.508: v21.21,8.38 21.46,8.13 32.77,8.13 v33.02,8.38 33.02,9.78 31.56,11.24 U5.1 | 54.13,42.29 53.49,41.66 | 50.16,39.88 R-T.2
  Top 0.61: v54.36,42.29 SWD.10
  Top 1.016: C31.1 R28.2 16.64,4.06 15.24,2.67 RST.2_1 | v21.21,8.38 20.45,9.14 D6.A
  Bottom 0.254: v54.86,20.45 54.86,23.62 55.63,24.38 55.63,30.73 54.36,32 54.36,33.66 55.12,34.42 55.12,41.53 v54.36,42.29
  Bottom 1.016: v21.21,5.84 v21.21,8.38 | v33.02,8.38 CON1.1
  Bottom 1.778: CON1.1 PLATFORM1.RST
TCK/SWCLK  (via drill 0.6)
  Top 0.254: U1.49 52.23,30.42 53.7,28.96 v53.72,28.96
  Top 0.66: v53.72,38.48 SWD.4
  Bottom 0.254: v53.72,28.96 53.34,29.34 53.34,38.1 v53.72,38.48
TDI  (via drill 0.6)
  Top 0.254: U1.50 51.49,29.92 v51.94,29.46
  Top 0.66: v54.23,40.89 54.36,41.02 SWD.8
  Bottom 0.254: v51.94,29.46 52.32,29.84 52.32,39.88 53.34,40.89 v54.23,40.89
TDO/SWO  (via drill 0.6)
  Top 0.254: U1.55 45.33,27.42 46.1,28.19 48.91,28.19 49.8,27.3 v52.83,27.3
  Top 0.66: v53.72,39.75 SWD.6
  Bottom 0.254: v52.83,27.3 52.83,38.99 53.34,39.5 53.59,39.75 v53.72,39.75
TMS/SWDIO  (via drill 0.6)
  Top 0.254: U1.46 47.41,31.45 47.88,30.99 52.38,30.99 53.14,30.23 v54.23,30.23
  Top 0.66: v54.23,37.34 54.36,37.21 SWD.2
  Bottom 0.254: v54.23,30.23 54.23,31.24 53.85,31.62 53.85,33.91 54.23,34.29 v54.23,37.34
TRST  (via drill 0.6)
  Top 0.254: U1.56 v46.1,26.92
  Top 0.508: v45.21,40.39 45.72,39.88 R-T.1
  Bottom 0.254: v46.1,26.92 46.1,31.11 46.48,31.5 46.48,35.43 45.21,36.7 v45.21,40.39
UEXT_#CS
  Top 0.254: 9.53,30.48 12.83,30.48 R10.1
  Top 0.381: 14.35,32 14.41,32.07 14.41,34.16 D10/D4.2
  Top 0.508: R10.1 14.35,32
  Top 1.016: UEXT.10 9.53,30.48
USB_P  (via drill 0.6)
  Top 0.254: U1.52 42.64,28.92 40.89,27.18 34.92,27.18 v34.16,26.42
  Top 0.508: v23.88,43.56 21.72,43.56
  Top 1.016: R2.1 21.72,43.56 R1.2
  Bottom 0.254: 24.89,43.56 25.27,43.18 26.42,43.18 27.69,44.45 29.72,44.45 30.73,45.47 35.56,45.47 37.34,43.69 37.34,37.34 34.54,34.54 34.54,26.8 v34.16,26.42
  Bottom 0.508: 24.89,43.56 v23.88,43.56
USB_SHIELD
  Top 1.016: USB.GND2 USB.GND1 2.41,48.26 2.41,38.36 USB.GND3 USB.GND4 8.13,38.36 8.13,39.62 9.78,41.27 C7.1
USBDM
  Top 0.254: U1.44 48.41,36.93 47.88,37.47 45.21,37.47 42.04,40.64 36.58,40.64 36.32,40.39 35.43,40.39 35.18,40.64 32.89,40.64 32.38,41.15 32.38,42.67 30.86,44.2 27.43,44.2 26.42,43.18 25.65,43.18 24.13,44.7 20.83,44.7 20.45,44.32 R3.1
  Top 1.016: R3.1 C9.1
USBDP
  Top 0.254: U1.45 47.91,36.67 47.62,36.96 44.96,36.96 41.78,40.13 36.83,40.13 36.58,39.88 35.18,39.88 34.92,40.13 32.64,40.13 31.88,40.89 31.88,42.47 30.66,43.69 27.69,43.69 26.67,42.67 23.11,42.67 22.73,42.29 22.73,41.66 22.48,41.4 21.06,41.4 19.66,42.8 R4.1
  Top 1.016: R4.1 C10.1 R5.1
VBAT  (via drill 0.6)
  Top 0.254: R34.2 55.37,13.34 55.37,11.43 59.69,7.11 59.69,4.32 59.18,3.81 31.88,3.81 30.48,2.41 v28.19,2.41
  Top 0.61: U3.3 25.78,13.52 C22.1
  Top 1.016: 28.57,13.46 FET1.3 | 28.57,13.46 C22.1 | v30.73,13.46 28.57,13.46
  Bottom 0.254: 15.24,2.03 16.76,0.51 26.29,0.51 v28.19,2.41 28.19,5.84 30.35,8 30.35,12.06 30.73,12.45 v30.73,13.46
  Bottom 1.016: LIPO_BAT.1 5.48,4.17 7.62,2.03 15.24,2.03
VCC  (via drill 0.6)
  Top 0.254: U1.1 46.41,20.19 44.2,20.19 43.31,21.08 43.31,22.61 43.18,22.73 43.37,22.92 U1.64 | U1.19 57.58,23.92 C5.2 | C3.2 57.09,30.42 U1.32 | U1.48 46.41,33.09 46.35,33.15 44.07,33.15 C4.2 | U6.5 10.34,43.56 v10.03,43.87
  Top 0.508: D6.C 16.59,8.51 12.95,8.51 12.57,8.13 10.79,8.13 v10.03,8.89 | 43.18,22.73 41.02,22.73 v41.02,22.99 | v40.64,36.7 40.64,36.96 | C4.2 43.31,32.13 42.16,30.99 v40.64,30.99 | 17.27,30.23 17.27,30.35 R10_E.2
  Top 0.66: v58.55,37.34 58.67,37.21 SWD.1
  Top 0.762: v10.03,45.85 C8.2 | 37.21,39.24 37.08,39.12 34.04,39.12 v33.91,39.24 | R11.1 11.43,33.4 12.32,32.51 12.32,32.13 v12.45,32
  Top 1.016: D6.C 16.64,9.1 R28.1 | 19.36,30.23 17.27,30.23 17.27,29.21 16.51,28.45 v16.26,28.45 14.86,28.45 | U5.2 33.46,10.86 v33.66,10.67 | v41.02,22.99 C6.2 | v40.64,36.7 R26.1 R27.1 | v58.55,25.53 58.55,24.89 C5.2 | v58.55,32.26 58.55,31.88 C3.2 | v35.56,8.64 v44.07,8.64 v47.62,8.64 | R11.1 R12.1 | 19.36,30.23 VR1.3 | 19.36,30.23 20.19,30.23 20.95,29.46 25.4,29.46 26.16,30.23 C26.1 26.16,30.48 C25.1 30.23,30.48 L2.1 30.48,30.25 31.11,29.61 v31.11,29.21 | T1.2 13.57,35.81 10.67,35.81 R12.1 | 10.67,36.45 R13.1 | 10.67,36.45 R14.1 12.45,36.45 v12.7,36.7 | R12.1 10.67,36.45 | 37.21,39.24 v40.64,39.24 | v33.91,39.24 31.11,39.24 L3.1 | v9.53,47.88 10.16,47.88 R30.1 | 14.86,28.45 R9.2 | 14.86,28.45 R8.2
  Bottom 0.762: 13.46,37.47 13.46,39.37 | 13.21,28.45 13.21,31.24 v12.45,32
  Bottom 1.016: v10.03,8.89 10.03,20.83 UEXT.1 12.7,23.5 12.7,27.94 13.21,28.45 v16.26,28.45 | 35.56,8.23 v35.56,8.64 35.56,8.76 v33.66,10.67 | v58.55,37.34 v58.55,32.26 v58.55,25.53 58.55,19.56 v47.62,8.64 | v44.07,8.64 44.07,19.94 v41.02,22.99 41.02,26.29 40.64,26.67 v40.64,30.99 v40.64,36.7 v40.64,39.24 | v9.53,47.88 10.03,47.37 v10.03,45.85 v10.03,43.87 10.03,42.8 13.46,39.37 | v12.7,36.7 13.46,37.47 | v31.11,29.21 32.13,30.23 32.13,35.69 33.91,37.47 v33.91,39.24
  Bottom 1.778: 35.56,8.23 CON1.2 PLATFORM1.3V3
VDD  (via drill 0.6)
  Top 0.254: U1.13 52.41,18.2 C2.2
  Top 0.762: L2.2 30.46,33.02 31.24,33.02 32.26,32 v35.94,32
  Top 1.016: C2.2 54.48,16.13 C1.2 v54.48,9.27 | L2.2 C27.1 30.23,35.69 C28.1 C30.1 25.4,35.69 24.51,34.8 20.32,34.8 20.04,35.08 VR2.3
  Bottom 0.254: 39.24,1.02 39.24,0.51 39.75,0.51 | 39.75,0.51 53.59,0.51 54.61,1.52 54.61,6.35 54.48,6.48 v54.48,9.27 | 39.75,0.51 39.75,1.02
  Bottom 1.016: 38.1,8.76 38.1,10.16 35.94,12.32 v35.94,32
  Bottom 1.27: 39.24,1.02 38.1,2.16 PLATFORM1.3V3A
  Bottom 1.778: PLATFORM1.3V3A CON1.3 38.1,8.76

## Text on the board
Top: 260 errors
Bottom: 146 errors
tPlace: 373 errors
tNames: OLIMEXINO-STM32 | Rev.E | 9-30VDC | + | + | WWW.OLIMEX.COM/DEV | CANH | CANL | GND | JUMPER | STATE | DESCRIPTION | UEXT_#CS is connected to D10 | D10/D4 | UEXT_#CS is connected to D4 | LED1_E is connected to D13 | LED1_E | LED1_E is not connected | LED2_E is connected to D3 | LED2_E | LED2_E is not connected | CAN termination is enabled | CAN_T | CAN termination is disabled | D23 is connected to EXT | D23_E | D23 is not connected to EXT | TRST and RESET are connected | R-T | TRST and RESET are separated
bNames: DIGITAL | CON4 | DIGITAL | CON3 | LED1 | LED2 | BUT | D14 | GND | D13 | D12 | D11 | D10 | D9 | D8 | D7 | D6 | D5 | D4 | D3 | D2 | D1 | D0 | USB | DESCRIPTION | STATE | JUMPER | UEXT_#CS is connected to D10 | UEXT_#CS is connected to D4 | D10/D4 | LED1_E is connected to D13 | LED1_E | LED1_E is not connected | LED2_E is connected to D3 | LED2_E is not connected | LED2_E | UEXT | CAN termination is enabled | CAN_T | CAN termination is disabled | D23 is connected to EXT | D23_E | D23 is not connected to EXT | TRST and RESET are connected | R-T | + | TRST and RESET are separated | Designed by: | - | www.olimex.com/dev | PWR_J | + | - | 9-30VDC | A5 | - | RST | 3V3 | 3V3A | GNDA | GND | VIN | A0 | A1 | A2 | A3 | A4 | + | RST | CANH | CANL | GND | 3.7V | - | LIPO_BAT | POWER | CON1 | ANALOG | CON2
213bmp: POLIGONI NA CIFROVOTO ZAHRANVANE I CHARGERA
